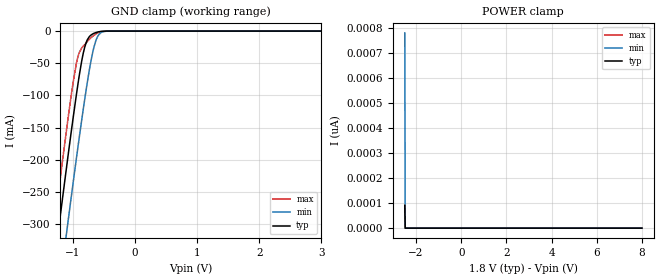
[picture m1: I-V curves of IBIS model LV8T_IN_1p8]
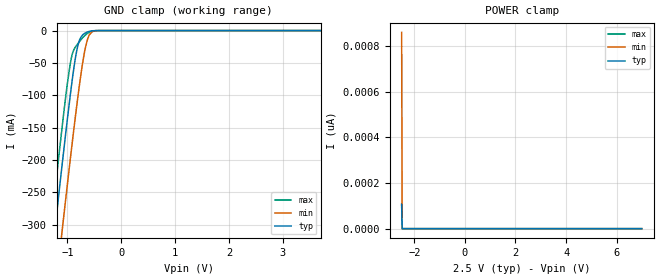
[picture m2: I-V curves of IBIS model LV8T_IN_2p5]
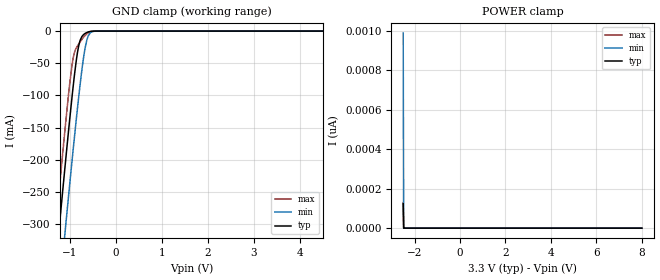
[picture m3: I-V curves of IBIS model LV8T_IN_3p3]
| TEXAS INSTRUMENTS INCORPORATED
| Standard Linear and Logic Group
| IBIS Model of SN74LV245A
| OCTAL BUS TRANSCEIVER WITH 3-STATE OUTPUTS
| SOIC 20-pin (DW), SOP 20-pin (NS), SSOP 20-pin (DB), TSSOP 20-pin (PW),
| TVSOP 20-pin (DGV), VQFN 20-pin (RKS) and SOT 20-pin (DGS) Packages
[IBIS Ver]   3.2
[Comment Char]  |_char
[File Name]   sn74lv8t245.ibs
[File Rev]   1.0
[Date]   Dec, 2022
[Source]   Data created from HSPICE simulations at TI.
[Notes]   The following is an IBIS list for the LV8T245.
|   The warning about non-monotonic V-I curves might be reported,
|   but it is nano ampere region and negligible.
|   The warning about AC Rising Endpoint might be reported,
|   but it is due to HSPICE issue and negligible.
[Disclaimer] Property of Texas Instruments Incorporated.  Unauthorized
   reproduction and/or distribution is strictly prohibited.
   This product is protected under copyright law.
   Created 2022, (C) Copyright 2022, Texas Instruments Inc.,
   All Rights Reserved.
   UNLESS THERE IS A SIGNED, WRITTEN AGREEMENT TO THE
   CONTRARY, TEXAS INSTRUMENTS () IS PROVIDING THE IBIS
   MODELS  AND WITHOUT ANY WARRANTY, EXPRESSED OR
   IMPLIED.  TI assumes no liability for:
   1) the accuracy of the IBIS models provided to your
   company;
   2) the proper functioning of these IBIS Models in your
   design or for any resulting applications; or
   3) infringement of patents, copyrights or intellectual
   property rights resulting from your use of these IBIS
   models.
   TI provides IBIS Models as a service to our customers.
   You and your company shall not distribute, sell or give
   these models to anyone else without prior written
   permission from TI.
   TI reserves the right to make changes to our products or
   to discontinue any semiconductor product or service
   without notice, and advises our customers to obtain the
   latest version of relevant information to verify, before
   placing orders, that the information being relied on is
   current.
   Please be aware that your receipt and use of the IBIS
   information provided shall serve as acceptance of these
   terms and conditions.  If you do not accept these terms,
   you should return or destroy the IBIS models and any
   other accompanying information immediately.
|   Component SN74LV8T245RKS
[Component]   SN74LV8T245RKS
[Manufacturer]   TI
[Package]   |VQFN, 20 pin RKS
|   typ   min   max
R_pkg   0.0928   0.0773   0.1056
L_pkg   1.6543nH   1.401nH   1.9974nH
C_pkg   0.2150pF   0.1865pF   0.2577pF
[Pin]   signal_name   model_name   R_pin   L_pin   C_pin
1   DIR   LV8T_IN   NA   NA   NA
2   A1   LV8T_OUT   NA   NA   NA
3   A2   LV8T_OUT   NA   NA   NA
4   A3   LV8T_OUT   NA   NA   NA
5   A4   LV8T_OUT   NA   NA   NA
6   A5   LV8T_OUT   NA   NA   NA
7   A6   LV8T_OUT   NA   NA   NA
8   A7   LV8T_OUT   NA   NA   NA
9   A8   LV8T_OUT   NA   NA   NA
10   GND   GND   NA   NA   NA
11   B8   LV8T_OUT   NA   NA   NA
12   B7   LV8T_OUT   NA   NA   NA
13   B6   LV8T_OUT   NA   NA   NA
14   B5   LV8T_OUT   NA   NA   NA
15   B4   LV8T_OUT   NA   NA   NA
16   B3   LV8T_OUT   NA   NA   NA
17   B2   LV8T_OUT   NA   NA   NA
18   B1   LV8T_OUT   NA   NA   NA
19   OE_NOT   LV8T_IN   NA   NA   NA
20   VCC   POWER   NA   NA   NA
|   Model Selector
[Model Selector]   LV8T_IN
LV8T_IN_1p8   1.8-V Vcc Input Model
LV8T_IN_2p5   2.5-V Vcc Input Model
LV8T_IN_3p3   3.3-V Vcc Input Model
LV8T_IN_5   5.0-V Vcc Input Model
[Model Selector]   LV8T_OUT
LV8T_OUT_1p8   1.8-V Vcc Output Model
LV8T_OUT_2p5   2.5-V Vcc Output Model
LV8T_OUT_3p3   3.3-V Vcc Output Model
LV8T_OUT_5   5.0-V Vcc Output Model
| Models and submodels in the file (8): LV8T_IN_1p8 (Input), LV8T_IN_2p5 (Input), LV8T_IN_3p3 (Input), LV8T_IN_5 (Input), LV8T_OUT_1p8 (I/O), LV8T_OUT_2p5 (I/O), LV8T_OUT_3p3 (I/O), LV8T_OUT_5 (I/O)
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|   Model LV8T_IN_33
[Model]   LV8T_IN_1p8
Model_type   Input
Vinl = 0.51
Vinh = 1.1
|   typ   min   max
C_comp   4.5pF   4.4pF   4.7pF
[Voltage Range]   1.8   1.65   2
[Temperature Range]   25   125   -40
[Power Clamp Reference]   1.8   1.65   2
[GND Clamp Reference]   0   0   0
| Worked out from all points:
|   GND clamp passes 1 mA (typ) near -0.58 V on its own axis
[GND Clamp]
|   Voltage   I(typ)   I(min)   I(max)
-2.5V     -1.312A    -1.405A    -1.262A
-1.313V   -372mA     -474.1mA   -313.7mA
-1.23V    -307.6mA   -410mA     -249mA
-1.145V   -244.1mA   -346.5mA   -185.5mA
-1.083V   -197.3mA   -299.5mA   -139.3mA
-935.5mV  -93.65mA   -192.4mA   -46.81mA
-830.5mV  -33.44mA   -120mA     -23.16mA
-778mV    -15.77mA   -86.16mA   -17.43mA
-715mV    -6.759mA   -49.81mA   -11.06mA
-620.5mV  -1.999mA   -12.46mA   -3.954mA
-431.5mV  -16.35uA   -111.6uA   -14.91uA
8V        0A         0A         0A
[POWER Clamp]
|   Voltage   I(typ)   I(min)   I(max)
-2.5V     90.39pA    780.9pA    92.69pA
-2.479V   0A         0A         0A
-2.469V   0A         0A         0A
8V        0A         0A         0A
[Model]   LV8T_IN_2p5
Model_type   Input
Vinl = 0.65
Vinh = 1.28
|   typ   min   max
C_comp   4.5pF   4.4pF   4.7pF
[Voltage Range]   2.5   2.25   2.75
[Temperature Range]   25   125   -40
[Power Clamp Reference]   2.5   2.25   2.75
[GND Clamp Reference]   0   0   0
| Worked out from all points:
|   GND clamp passes 1 mA (typ) near -0.58 V on its own axis
[GND Clamp]
|   Voltage   I(typ)   I(min)   I(max)
-2.5V     -1.312A    -1.405A    -1.262A
-1.313V   -372mA     -474.1mA   -313.7mA
-1.23V    -307.6mA   -410mA     -249mA
-1.083V   -197.3mA   -299.5mA   -139.3mA
-935.5mV  -93.65mA   -192.4mA   -46.81mA
-830.5mV  -33.44mA   -120mA     -23.16mA
-767.5mV  -13.53mA   -79.7mA    -16.3mA
-694mV    -5.257mA   -39.32mA   -9.204mA
-631mV    -2.338mA   -15.21mA   -4.578mA
-547mV    -490uA     -2.342mA   -941uA
-431.5mV  -16.35uA   -111.6uA   -14.91uA
6.992V    0A         0A         0A
[POWER Clamp]
|   Voltage   I(typ)   I(min)   I(max)
-2.5V     105.6pA    858.9pA    109.1pA
-2.479V   0A         0A         0A
-2.469V   0A         0A         0A
6.992V    0A         0A         0A
[Model]   LV8T_IN_3p3
Model_type   Input
Vinl = 0.75
Vinh = 1.45
|   typ   min   max
C_comp   4.5pF   4.4pF   4.7pF
[Voltage Range]   3.3   3   3.6
[Temperature Range]   25   125   -40
[Power Clamp Reference]   3.3   3   3.6
[GND Clamp Reference]   0   0   0
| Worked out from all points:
|   GND clamp passes 1 mA (typ) near -0.58 V on its own axis
[GND Clamp]
|   Voltage   I(typ)   I(min)   I(max)
-2.5V     -1.312A    -1.405A    -1.262A
-1.313V   -372mA     -474.1mA   -313.7mA
-1.23V    -307.6mA   -410mA     -249mA
-1.145V   -244.1mA   -346.5mA   -185.5mA
-1.083V   -197.3mA   -299.5mA   -139.3mA
-935.5mV  -93.65mA   -192.4mA   -46.81mA
-830.5mV  -33.44mA   -120mA     -23.16mA
-778mV    -15.77mA   -86.16mA   -17.43mA
-715mV    -6.759mA   -49.81mA   -11.06mA
-620.5mV  -1.999mA   -12.46mA   -3.954mA
-431.5mV  -16.35uA   -111.6uA   -14.91uA
8V        0A         0A         0A
[POWER Clamp]
|   Voltage   I(typ)   I(min)   I(max)
-2.5V     124pA      988.9pA    129.3pA
-2.479V   0A         0A         0A
-2.469V   0A         0A         0A
8V        0A         0A         0A
